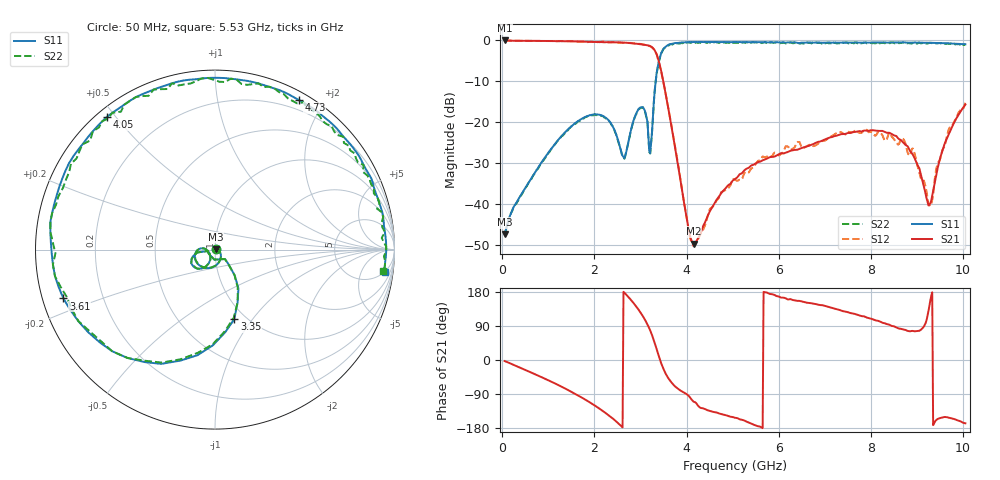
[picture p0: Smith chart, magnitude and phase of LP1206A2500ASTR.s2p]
!Instrument:	"HEWLETT PACKARD,8720ES,US39172150,7.62 "
!	LP1206	High	Performance	Low	Pass	Filters
!	P/N	LP1206A2500ASTR	6	May	2019
#	MHz	S	dB	R	50
!	Frq	S11(dB)	S11(deg)	S21(dB)	S21(deg)	S12(dB)	S12(deg)	S22(dB)	S22(deg)
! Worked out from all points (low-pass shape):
!   501 points, 50 MHz to 10.05 GHz, reference 50 ohm
!   highest |S21| = 0.00 dB at 50 MHz (marker M1); lowest = -49.7 dB at 4.15 GHz (marker M2)
!   |S21| within 3 dB of the highest: start of sweep to 3.334 GHz
!   lowest |S11| = -47.5 dB at 50 MHz (marker M3), VSWR 1.01, Z = 50.3 + j0.298 ohm
!   |S11| at or under -10 dB: start of sweep to 3.329 GHz
!   |S22| runs from -47.5 to -0.4 dB; largest |S21 - S12| = 0.032
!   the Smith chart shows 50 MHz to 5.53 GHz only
!   S11 on the Smith chart (normalised r, x): 50 MHz: 1.01, +0.01; 3.35 GHz: 0.89, -0.82; 3.61 GHz: 0.06, -0.16; 4.05 GHz: 0.03, +0.47; 4.73 GHz: 0.09, +1.70; 5.53 GHz: 5, -14
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50  -47.48 44.6  0.00 -2.8  -0.07 -2.4  -47.48 44.6
1730  -19.13 -111.0  -0.27 -99.5  -0.28 -99.6  -19.33 -111.2
2210  -18.65 -163.8  -0.44 -137.0  -0.27 -137.3  -18.85 -164.0
2710  -26.30 -122.1  -0.58 169.7  -0.60 169.3  -26.30 -122.2
3010  -16.33 -142.1  -0.96 123.3  -0.87 123.2  -16.53 -142.1
3210  -27.58 -143.2  -1.37 77.9  -1.46 77.2  -27.68 -143.4
3350  -7.91 -74.5  -3.34 28.9  -3.44 26.2  -8.11 -74.5
3390  -5.46 -91.3  -4.82 12.8  -4.99 10.5  -5.56 -91.4
3610  -1.04 -162.1  -17.09 -49.4  -16.98 -51.5  -1.24 -162.2
4050  -0.41 129.2  -46.57 -95.3  -47.05 -92.7  -0.51 129.2
4150  -0.38 117.4  -49.71 -109.9  -50.35 -104.0  -0.38 117.3
4730  -0.39 60.8  -37.74 -142.0  -37.71 -140.0  -0.59 60.7
5050  -0.38 33.1  -33.93 -152.4  -34.07 -154.5  -0.58 33.0
5530  -0.42 -7.4  -29.89 -174.0  -29.76 -167.5  -0.52 -7.4
6210  -0.47 -64.5  -27.23 159.7  -26.09 154.8  -0.47 -64.6
6730  -0.53 -108.7  -25.44 149.2  -25.71 147.0  -0.53 -108.8
7570  -0.53 179.2  -22.58 123.6  -22.47 122.7  -0.53 179.2
8390  -0.50 108.2  -22.59 93.5  -22.66 102.1  -0.60 108.0
8930  -0.52 60.4  -28.42 76.2  -27.10 79.3  -0.72 60.2
9290  -0.57 27.3  -39.87 157.8  -40.53 152.4  -0.57 27.1
9670  -0.72 -9.0  -23.43 -151.6  -22.53 -149.6  -0.72 -9.0
10050  -0.95 -46.8  -15.71 -167.1  -15.25 -165.5  -1.15 -46.8
